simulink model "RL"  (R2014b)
settings: Solver=ode45  StartTime=0.0  StopTime=10.0  RelTol=1e-3
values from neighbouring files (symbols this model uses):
  E = sqrt(Ex.^2+Ey.^2+eps)    [ElectDipole.m]
  R = zeros(N,N)    [romberg.m]
undefined symbols (not defined in the file or in its folder): L

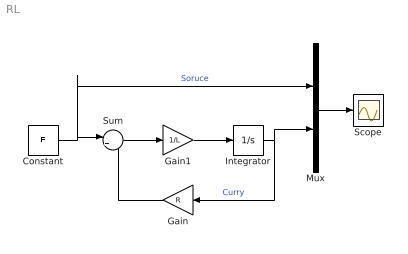
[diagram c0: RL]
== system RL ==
  Constant : Constant  Value=E
  Gain : Gain  Gain=R
  Gain1 : Gain  Gain=1/L
  Integrator : Integrator
  Mux : Mux  Inputs=2
  Scope : Scope
  Sum : Sum  Inputs=|+-
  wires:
  Constant/1 -> Mux/1, Sum/1  "Soruce"
  Gain/1 -> Sum/2
  Sum/1 -> Gain1/1
  Gain1/1 -> Integrator/1
  Integrator/1 -> Mux/2, Gain/1  "Curry"
  Mux/1 -> Scope/1
